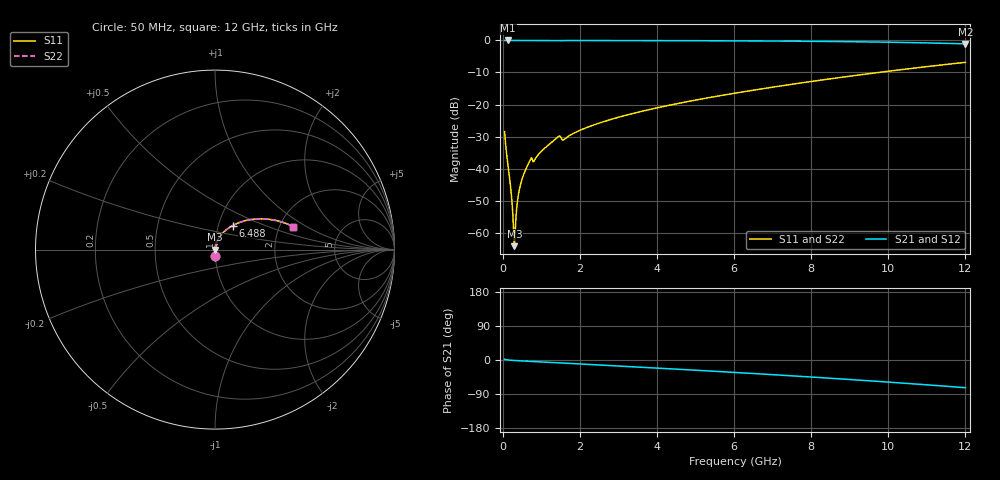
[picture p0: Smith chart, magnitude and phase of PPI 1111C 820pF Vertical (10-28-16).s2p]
# GHz S MA R 50
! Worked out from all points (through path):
!   1601 points, 50 MHz to 12 GHz, reference 50 ohm
!   highest |S21| = 0.00 dB at 139.6 MHz (marker M1); lowest = -1.1 dB at 12 GHz (marker M2)
!   group delay of S21, straight-line fit = 16.7 ps
!   lowest |S11| = -64.2 dB at 303.9 MHz (marker M3), VSWR 1.00, Z = 50.1 - j0.00168 ohm
!   |S11| at or under -10 dB: start of sweep to 9.743 GHz
!   |S22| runs from -64.2 to -6.8 dB; largest |S21 - S12| = 0
!   S11 on the Smith chart (normalised r, x): 50 MHz: 1.00, -0.08; 6.488 GHz: 1.17, +0.32; 12 GHz: 2.38, +0.77
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0.05  0.03771 -87.6  0.999 2.0  0.999 2.0  0.03771 -87.6
0.08734375  0.02038 -88.1  0.9994 0.8  0.9994 0.8  0.02038 -88.1
0.139625  0.01098 -87.6  0.9995 0.1  0.9995 0.1  0.01098 -87.6
0.2068437  0.005073 -84.6  0.9994 -0.6  0.9994 -0.6  0.005073 -84.6
0.2665938  0.001785 -72.0  0.9994 -1.0  0.9994 -1.0  0.001785 -72.0
0.3039375  0.0006152 -1.6  0.9994 -1.2  0.9994 -1.2  0.0006152 -1.6
0.3412812  0.001622 65.0  0.9993 -1.5  0.9993 -1.5  0.001622 65.0
0.4010313  0.00368 77.3  0.9993 -1.9  0.9993 -1.9  0.00368 77.3
0.46825  0.005818 80.4  0.9992 -2.2  0.9992 -2.2  0.005818 80.4
0.557875  0.008495 81.6  0.9991 -2.8  0.9991 -2.8  0.008495 81.6
0.6997813  0.01307 80.1  0.9985 -3.6  0.9985 -3.6  0.01307 80.1
0.8342188  0.01382 78.9  0.9982 -4.2  0.9982 -4.2  0.01382 78.9
1.431719  0.03118 76.0  0.996 -7.6  0.996 -7.6  0.03118 76.0
1.596031  0.02851 74.6  0.9959 -8.1  0.9959 -8.1  0.02851 74.6
2.044156  0.04055 77.1  0.9975 -10.7  0.9975 -10.7  0.04055 77.1
2.888125  0.06047 73.1  0.9963 -15.2  0.9963 -15.2  0.06047 73.1
4.038312  0.08968 67.2  0.9937 -21.5  0.9937 -21.5  0.08968 67.2
6.025  0.1504 56.2  0.9857 -32.8  0.9857 -32.8  0.1504 56.2
6.488062  0.167 53.5  0.9829 -35.5  0.9829 -35.5  0.167 53.5
8.019156  0.2296 44.2  0.9696 -45.0  0.9696 -45.0  0.2296 44.2
10.01331  0.3314 30.9  0.939 -58.4  0.939 -58.4  0.3314 30.9
12  0.4551 16.3  0.8849 -73.1  0.8849 -73.1  0.4551 16.3
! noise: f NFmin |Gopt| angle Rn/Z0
0.05  0.0003805  0.8688  0.2264  0.0006238
1.372  0.005173  0.7522  5.547  0.004201
2.701  0.006633  0.6447  10.7  0.003506
4.031  0.008908  0.6156  15.72  0.004234
5.36  0.01115  0.6002  20.58  0.004982
6.682  0.0134  0.5933  25.26  0.005773
8.012  0.01576  0.5929  29.79  0.006659
9.341  0.01827  0.598  34.17  0.007687
10.67  0.02102  0.608  38.41  0.008917
12  0.02409  0.6223  42.53  0.01043
